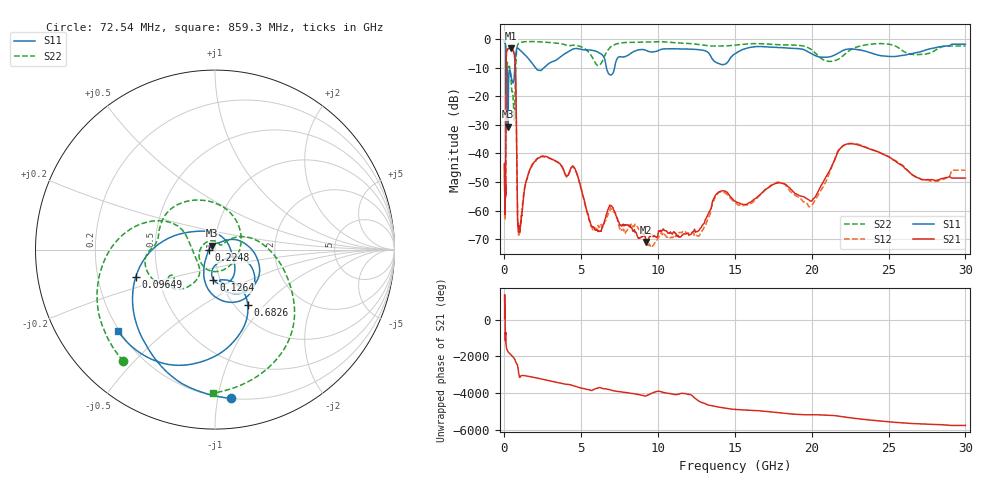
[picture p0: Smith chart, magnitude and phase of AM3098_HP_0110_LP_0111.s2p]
! Date/Time: Thu, Feb 28, 2019 8:37 AM
! Network Analyzer: Agilent Technologies E8364B Rev: A.07.50.67
! Sweep from 0.010 to 30.000 GHz, 1601 Points, Sweep Type: LOG
! Power Supply: 5.022 V, 0.002 A
# Hz S DB R 50
!freq MagS11 AngS11 MagS21 AngS21 MagS12 AngS12 MagS22 AngS22
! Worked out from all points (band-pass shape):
!   1601 points, 10 MHz to 30 GHz, reference 50 ohm
!   highest |S21| = -3.10 dB at 399.6 MHz (marker M1); lowest = -71.0 dB at 9.21 GHz (marker M2)
!   |S21| within 3 dB of the highest: 117.5 MHz to 660.2 MHz (542.7 MHz wide, 140 % of centre)
!   lowest |S11| = -30.6 dB at 230.5 MHz (marker M3), VSWR 1.06, Z = 48.1 + j2.15 ohm
!   |S11| at or under -10 dB: 175.7 MHz to 671.5 MHz (495.8 MHz wide, 117 % of centre); 2.039 GHz to 2.55 GHz (511.1 MHz wide, 22.3 % of centre); 6.64 GHz to 7.165 GHz (524.5 MHz wide, 7.6 % of centre)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
!   |S22| runs from -28.3 to -0.5 dB; largest |S21 - S12| = 0.012
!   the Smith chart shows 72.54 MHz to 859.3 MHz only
!   S11 on the Smith chart (normalised r, x): 72.54 MHz: 0.20, -1.09; 96.49 MHz: 0.37, -0.14; 126.4 MHz: 0.93, -0.32; 224.8 MHz: 0.93, -0.00; 682.6 MHz: 1.14, -0.80; 859.3 MHz: 0.19, -0.35
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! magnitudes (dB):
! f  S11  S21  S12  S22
! 10 MHz  -0.4  -43.6  -44.8  -0.5
! 38.04 MHz  -0.5  -59.0  -62.9  -0.9
! 72.54 MHz  -1.6  -53.8  -51.3  -1.9
! 83.04 MHz  -2.5  -51.1  -53.8  -2.7
! 96.49 MHz  -6.6  -25.7  -25.7  -7.4
! 126.4 MHz  -15.5  -5.1  -5.1  -9.9
! 144.7 MHz  -18.3  -4.0  -4.0  -11.1
! 183.1 MHz  -10.6  -3.7  -3.7  -8.0
! 224.8 MHz  -29.0  -3.3  -3.2  -9.3
! 230.5 MHz  -30.6  -3.2  -3.2  -9.5
! 399.6 MHz  -12.0  -3.1  -3.1  -12.1
! 550.5 MHz  -15.2  -3.8  -3.7  -19.3
! 682.6 MHz  -9.0  -7.5  -7.5  -20.6
! 859.3 MHz  -3.0  -63.8  -63.6  -1.9
! 2.084 GHz  -10.3  -42.1  -42.2  -0.8
! 4.503 GHz  -3.3  -44.7  -44.7  -2.0
! 5.841 GHz  -3.9  -66.2  -66.7  -7.5
! 7.926 GHz  -5.9  -65.1  -67.2  -1.0
! 9.21 GHz  -3.9  -71.0  -70.3  -0.9
! 19.9 GHz  -4.7  -56.7  -58.7  -3.3
! 22.67 GHz  -3.4  -36.6  -36.5  -3.2
! 30 GHz  -1.7  -48.6  -45.9  -2.3
